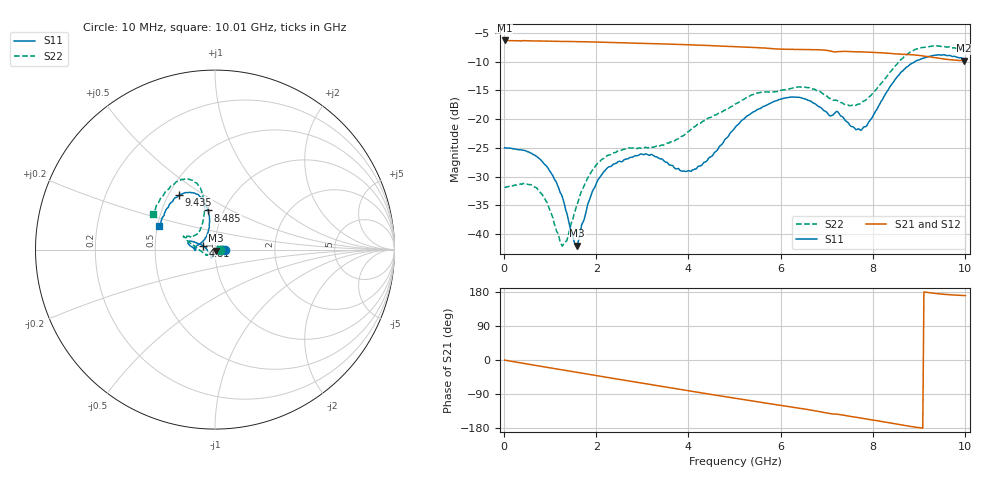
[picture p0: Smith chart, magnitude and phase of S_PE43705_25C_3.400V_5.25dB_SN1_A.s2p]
! Device ID: PE43705
! Serial: 1
! Insertion: A
! Impedance: 50 ohm
! Temp: 25C
! VDD: 3.400V
! Attenuation Step: 5.25dB
#  Hz  S  RI  R  50
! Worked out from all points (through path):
!   401 points, 10 MHz to 10.01 GHz, reference 50 ohm
!   highest |S21| = -6.29 dB at 10 MHz (marker M1); lowest = -9.8 dB at 9.985 GHz (marker M2)
!   group delay of S21, straight-line fit = 54.2 ps
!   lowest |S11| = -42.1 dB at 1.585 GHz (marker M3), VSWR 1.02, Z = 50.4 - j0.676 ohm
!   |S11| at or under -10 dB: start of sweep to 8.908 GHz
!   |S22| runs from -42.1 to -7.2 dB; largest |S21 - S12| = 0.0041
!   S11 on the Smith chart (normalised r, x): 10 MHz: 1.12, -0.00; 4.81 GHz: 0.88, +0.03; 8.485 GHz: 0.84, +0.39; 9.435 GHz: 0.57, +0.40; 10.01 GHz: 0.51, +0.15
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1e7  0.0563 -6.4e-05  0.4845 -0.00245  0.485 -0.00209  0.0256 3.96e-05
7.35e8  0.0423 0.0185  0.4621 -0.1267  0.4622 -0.1264  0.0155 0.0185
1.26e9  0.0201 0.00686  0.4272 -0.2088  0.4275 -0.2085  -0.00379 0.00684
1.485e9  0.00924 -0.00271  0.4079 -0.2416  0.408 -0.2416  -0.0129 -0.00204
1.585e9  0.00417 -0.0067  0.398 -0.2553  0.3982 -0.2552  -0.0171 -0.00612
1.685e9  0.00038 -0.0121  0.3883 -0.2688  0.3884 -0.2688  -0.0216 -0.0105
1.935e9  -0.00845 -0.0229  0.3614 -0.3008  0.3614 -0.3006  -0.0309 -0.0201
2.235e9  -0.0149 -0.0344  0.3253 -0.3354  0.3255 -0.3352  -0.0385 -0.029
2.935e9  -0.0207 -0.0444  0.2293 -0.3976  0.23 -0.3975  -0.0478 -0.0293
3.36e9  -0.0194 -0.0413  0.1666 -0.4211  0.1672 -0.4206  -0.0513 -0.0269
4.085e9  -0.0329 -0.0147  0.0559 -0.4391  0.0565 -0.439  -0.0838 -0.0058
4.81e9  -0.0647 0.0197  -0.0532 -0.4273  -0.0525 -0.4273  -0.1186 0.0218
5.01e9  -0.0792 0.029  -0.0815 -0.4196  -0.0809 -0.4198  -0.1314 0.0311
5.985e9  -0.1411 0.0474  -0.2007 -0.3549  -0.1988 -0.3554  -0.1641 0.066
6.685e9  -0.1386 0.0211  -0.274 -0.2955  -0.2738 -0.2952  -0.1669 0.0754
7.71e9  -0.0624 0.0525  -0.3424 -0.1773  -0.3418 -0.178  -0.0846 0.1057
8.36e9  -0.0312 0.1853  -0.363 -0.0918  -0.3616 -0.0934  -0.0601 0.2457
8.485e9  -0.0383 0.2184  -0.3636 -0.0734  -0.3622 -0.0756  -0.0649 0.2832
8.91e9  -0.0899 0.3036  -0.3617 -0.02  -0.3597 -0.0203  -0.1215 0.3841
9.435e9  -0.1993 0.3042  -0.3373 0.0313  -0.3363 0.0314  -0.2219 0.3715
9.985e9  -0.302 0.1422  -0.3181 0.0551  -0.319 0.0547  -0.3362 0.2117
1.001e10  -0.3097 0.133  -0.3188 0.0564  -0.3202 0.0551  -0.3444 0.2009
